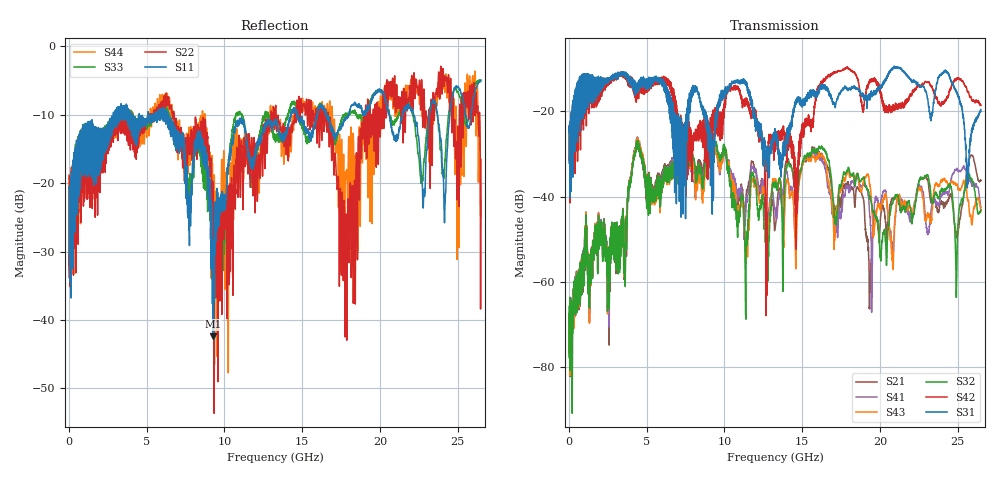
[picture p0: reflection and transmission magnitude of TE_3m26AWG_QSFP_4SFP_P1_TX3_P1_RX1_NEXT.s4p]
!Agilent Technologies,N5222A,MY51421691,A.10.00.00
!Agilent N5222A: A.10.00.00
!Date: Friday, January 30, 2015 12:33:58
!Correction: S11(Full 4 Port(1,2,3,4))
!S12(Full 4 Port(1,2,3,4))
!S13(Full 4 Port(1,2,3,4))
!S14(Full 4 Port(1,2,3,4))
!S21(Full 4 Port(1,2,3,4))
!S22(Full 4 Port(1,2,3,4))
!S23(Full 4 Port(1,2,3,4))
!S24(Full 4 Port(1,2,3,4))
!S31(Full 4 Port(1,2,3,4))
!S32(Full 4 Port(1,2,3,4))
!S33(Full 4 Port(1,2,3,4))
!S34(Full 4 Port(1,2,3,4))
!S41(Full 4 Port(1,2,3,4))
!S42(Full 4 Port(1,2,3,4))
!S43(Full 4 Port(1,2,3,4))
!S44(Full 4 Port(1,2,3,4))
!S4P File: Measurements: <S11,S12,S13,S14>,
!<S21,S22,S23,S24>,
!<S31,S32,S33,S34>,
!<S41,S42,S43,S44>:
# Hz S  dB  R 50.0
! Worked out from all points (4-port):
!   2650 points, 10 MHz to 26.5 GHz, reference 50 ohm
!   strongest paths, dB at 10 MHz, 6.63 GHz, 13.26 GHz, 19.88 GHz, 26.5 GHz:
!     S31: -24.9, -17.8, -24.7, -15.3, -19.6
!     S42: -24.7, -16.1, -29.4, -13.4, -18.5
!     S32: -65.7, -31.9, -36.6, -46.0, -43.1
!     S43: -76.7, -32.3, -35.8, -41.7, -43.5
!     S41: -70.8, -31.3, -42.8, -40.9, -42.5
!     S21: -67.1, -30.9, -47.0, -47.6, -36.2
!   lowest |S11| = -42.4 dB at 9.27 GHz (marker M1), VSWR 1.02, Z = 50 + j0.759 ohm
!   |S11| at or under -10 dB: start of sweep to 2.858 GHz; 6.4 GHz to 14.26 GHz (7.857 GHz wide, 76.1 % of centre); 16.59 GHz to 17.99 GHz (1.395 GHz wide, 8.07 % of centre)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
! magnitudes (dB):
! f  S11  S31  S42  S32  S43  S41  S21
! 10 MHz  -20.8  -24.9  -24.7  -65.7  -76.7  -70.8  -67.1
! 4.36 GHz  -12.3  -15.1  -16.8  -29.0  -28.6  -28.5  -28.9
! 9.27 GHz  -42.4  -27.7  -23.3  -27.1  -28.6  -27.2  -26.2
! 11.4 GHz  -13.3  -14.0  -17.2  -51.6  -50.0  -41.6  -39.5
! 12.68 GHz  -11.2  -29.3  -45.3  -52.5  -41.2  -42.1  -49.6
! 19.36 GHz  -8.5  -17.4  -12.7  -40.3  -37.2  -44.7  -61.5
! 26.5 GHz  -4.9  -19.6  -18.5  -43.1  -43.5  -42.5  -36.2
